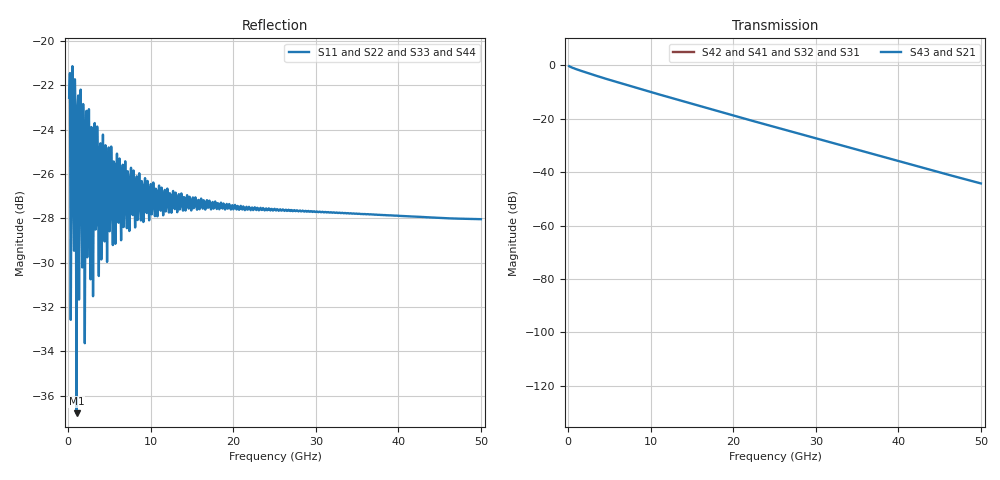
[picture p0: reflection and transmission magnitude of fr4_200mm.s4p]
! Touchstone Ver. 1.0
! Number of ports is 4
! port1 ->  port2
! port3 ->  port4
# Hz	S	RI	R	50.000000
! SCATTERING PARAMETERS  :
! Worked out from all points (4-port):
!   500 points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, 100 MHz to 50 GHz, reference 50 ohm
!   strongest paths, dB at 100 MHz, 12.6 GHz, 25.1 GHz, 37.6 GHz, 50 GHz:
!     S43: -0.3, -12.3, -23.1, -33.8, -44.2
!     S21: -0.3, -12.3, -23.1, -33.8, -44.2
!     S42: -, -, -, -, -
!     S41: -, -, -, -, -
!     S32: -, -, -, -, -
!     S31: -, -, -, -, -
!   lowest |S11| = -36.8 dB at 1 GHz (marker M1), VSWR 1.03, Z = 48.6 - j0.346 ohm
!   |S11| at or under -10 dB: start of sweep to end of sweep
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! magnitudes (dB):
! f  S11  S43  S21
! 100 MHz  -22.6  -0.3  -0.3
! 800 MHz  -21.7  -1.3  -1.3
! 1 GHz  -36.8  -1.5  -1.5
! 1.2 GHz  -22.5  -1.7  -1.7
! 1.3 GHz  -31.7  -1.8  -1.8
! 2.2 GHz  -23.2  -2.8  -2.8
! 50 GHz  -28.0  -44.2  -44.2
